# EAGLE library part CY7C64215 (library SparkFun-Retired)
Cypress PSOC uC with USB SparkFun Products None
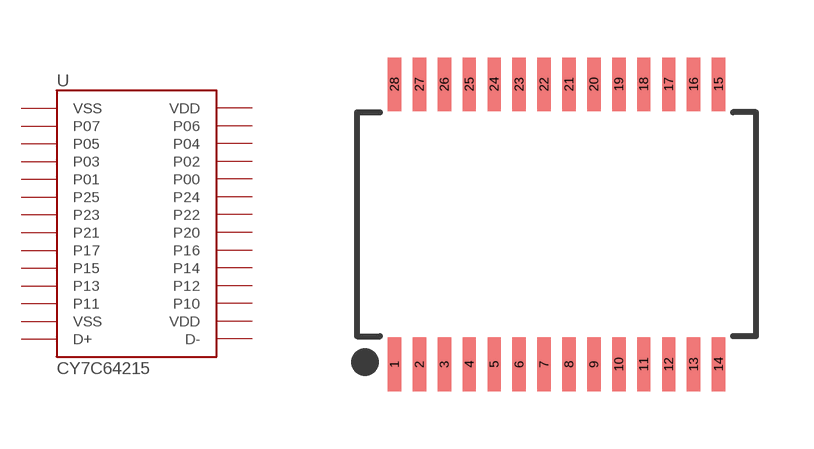
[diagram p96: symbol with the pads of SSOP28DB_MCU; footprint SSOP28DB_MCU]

Designator prefix -

## CY7C64215  [SSOP28DB_MCU]
1  VSS
2  P07
3  P05
4  P03
5  P01
6  P25
7  P23
8  P21
9  P17
10  P15
11  P13
12  P11
13  VSS
14  D+
15  D-
16  VDD
17  P10
18  P12
19  P14
20  P16
21  P20
22  P22
23  P24
24  P00
25  P02
26  P04
27  P06
28  VDD

## Footprint SSOP28DB_MCU (pad centres in mm)
Small Shrink Outline Package
smd 0.348 x 1.397: 1 -4.225,-3.656; 2 -3.575,-3.656; 3 -2.925,-3.656; 4 -2.275,-3.656; 5 -1.625,-3.656; 6 -0.975,-3.656; 7 -0.325,-3.656; 8 0.325,-3.656; 9 0.975,-3.656; 10 1.625,-3.656; 11 2.275,-3.656; 12 2.925,-3.656; 13 3.575,-3.656; 14 4.225,-3.656; 15 4.225,3.656; 16 3.575,3.656; 17 2.925,3.656; 18 2.275,3.656; 19 1.625,3.656; 20 0.975,3.656; 21 0.325,3.656; 22 -0.325,3.656; 23 -0.975,3.656; 24 -1.625,3.656; 25 -2.275,3.656; 26 -2.925,3.656; 27 -3.575,3.656; 28 -4.225,3.656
